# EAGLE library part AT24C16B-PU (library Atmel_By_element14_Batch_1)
Two-wire Serial EEPROM
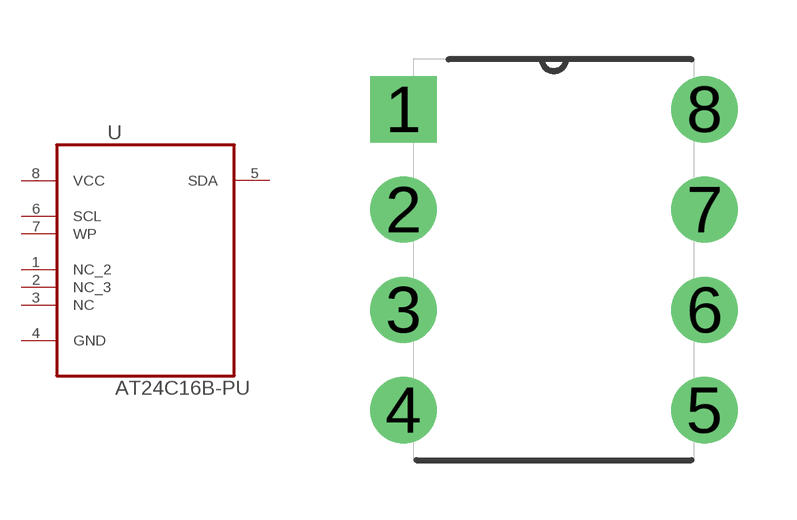
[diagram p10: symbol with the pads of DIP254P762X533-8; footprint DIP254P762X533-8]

Designator prefix U

## AT24C16B-PU (MPN: AT24C16B-PU; OC_FARNELL: 1362650; OC_NEWARK: 50M3323; PACKAGE: PDIP-8; SUPPLIER: Atmel)  [DIP254P762X533-8]
1  NC_2  nc
2  NC_3  nc
3  NC  nc
4  GND  pas
5  SDA
6  SCL  in
7  WP  in
8  VCC  pwr

## Footprint DIP254P762X533-8 (pad centres in mm)
drill 1.118 square: 1 -7.62,7.62
drill 1.118: 2 -7.62,5.08; 3 -7.62,2.54; 4 -7.62,0; 5 0,0; 6 0,2.54; 7 0,5.08; 8 0,7.62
